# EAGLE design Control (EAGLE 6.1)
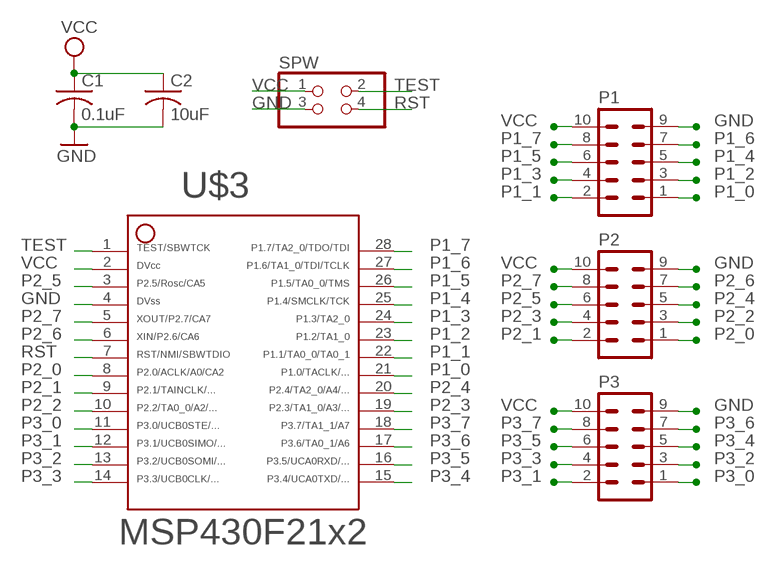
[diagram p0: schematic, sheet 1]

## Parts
C1  0.1uF  C-USC0603K  [C0603K]
C2  10uF  C-USC0603K  [C0603K]
P1  MA05-2  [MA05-2]
P2  MA05-2  [MA05-2]
P3  MA05-2  [MA05-2]
SPW  PINHD-2X2  [2X02]
U$3  F21X2---PW28  [PW28]

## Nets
GND: C1.2 C2.2 P1.9 P2.9 P3.9 SPW.3 U$3.4
P1_0: P1.1 U$3.21
P1_1: P1.2 U$3.22
P1_2: P1.3 U$3.23
P1_3: P1.4 U$3.24
P1_4: P1.5 U$3.25
P1_5: P1.6 U$3.26
P1_6: P1.7 U$3.27
P1_7: P1.8 U$3.28
P2_0: P2.1 U$3.8
P2_1: P2.2 U$3.9
P2_2: P2.3 U$3.10
P2_3: P2.4 U$3.19
P2_4: P2.5 U$3.20
P2_5: P2.6 U$3.3
P2_6: P2.7 U$3.6
P2_7: P2.8 U$3.5
P3_0: P3.1 U$3.11
P3_1: P3.2 U$3.12
P3_2: P3.3 U$3.13
P3_3: P3.4 U$3.14
P3_4: P3.5 U$3.15
P3_5: P3.6 U$3.16
P3_6: P3.7 U$3.17
P3_7: P3.8 U$3.18
RST: SPW.4 U$3.7
TEST: SPW.2 U$3.1
VCC: C1.1 C2.1 P1.10 P2.10 P3.10 SPW.1 U$3.2

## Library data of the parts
C1 C2 = rcl:C-US: CAPACITOR, American symbol
P1-P3 = con-lstb:MA05-2: PIN HEADER; OC_FARNELL: unknown; OC_NEWARK: unknown
SPW = pinhead:PINHD-2X2: PIN HEADER
U$3 = TI_MSP430_v16:F21X2---PW28: *** MSP430F21x2 *** PW28

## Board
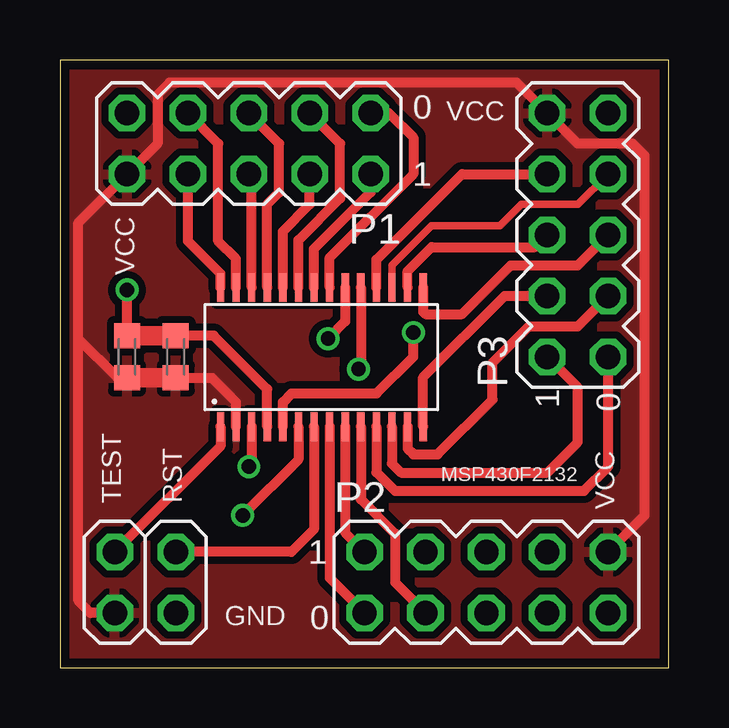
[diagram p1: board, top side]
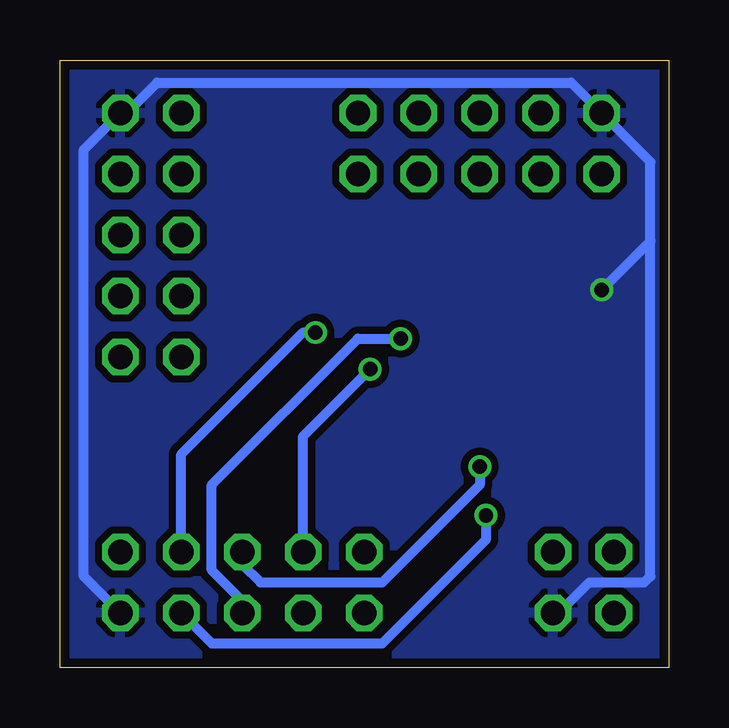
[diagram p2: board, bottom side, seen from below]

Size 25.38 x 25.32 mm. Coordinates in mm from the lower left corner, seen from the top.
Outline: 0,0 25.38,0 25.38,25.32 0,25.32 0,0
Copper layers (1*16): Top 0.0356mm / dielectric 1.5011mm / Bottom 0.0356mm
Design rules: minimum track width 6mil, minimum drill 13mil, track to track 6mil, track to pad 6mil, pad to pad 6mil, via to via 6mil, smd to smd 6mil, copper to edge 15mil, drill to drill 6mil, minimum pad ring 7mil, minimum via ring 7mil, stop-mask expansion 4mil, vias tented up to drill 0mil, thermal gap 10mil

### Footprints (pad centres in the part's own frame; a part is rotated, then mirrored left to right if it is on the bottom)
C0603K = smd 1.05 x 1.08: 1 -0.875,0; 2 0.875,0
MA05-2 = drill 1.016 octagon: 1 -5.08,-1.27; 2 -5.08,1.27; 3 -2.54,-1.27; 4 -2.54,1.27; 5 0,-1.27; 6 0,1.27; 7 2.54,-1.27; 8 2.54,1.27; 9 5.08,-1.27; 10 5.08,1.27
2X02 = drill 1.016 octagon: 1 -1.27,-1.27; 2 -1.27,1.27; 3 1.27,-1.27; 4 1.27,1.27
PW28 = smd 0.3 x 1.2: 1 -4.229,-2.908; 2 -3.579,-2.908; 3 -2.929,-2.908; 4 -2.279,-2.908; 5 -1.629,-2.908; 6 -0.979,-2.908; 7 -0.329,-2.908; 8 0.321,-2.908; 9 0.971,-2.908; 10 1.621,-2.908; 11 2.271,-2.908; 12 2.921,-2.908; 13 3.571,-2.908; 14 4.221,-2.908; 15 4.221,2.892; 16 3.571,2.892; 17 2.921,2.892; 18 2.271,2.892; 19 1.621,2.892; 20 0.971,2.892; 21 0.321,2.892; 22 -0.329,2.892; 23 -0.979,2.892; 24 -1.629,2.892; 25 -2.279,2.892; 26 -2.929,2.892; 27 -3.579,2.892; 28 -4.229,2.892

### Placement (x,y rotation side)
C1  4.83,12.95 90 top
C2  2.79,12.95 90 top
P1  7.87,21.84 180 top
P2  17.78,3.56 0 top
P3  21.59,18.03 90 top
SPW  3.56,3.56 0 top
U$3  10.92,12.95 0 top

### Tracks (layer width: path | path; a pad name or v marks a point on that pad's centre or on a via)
GND  (via drill 0.6)
  Top 0.406: U$3.4 8.64,11.61 6.41,13.84 4.84,13.84 C1.2 | C2.2 v2.79,15.75
  Top 0.813: C1.2 C2.2
  Bottom 0.406: P2.9 24.38,3.81 24.38,21.59 P3.9 22.61,23.11 21.34,24.38 4.06,24.38 P1.9 0.76,21.08 0.76,17.78 | SPW.3 4.57,2.29 3.3,3.56 1.02,3.56 0.76,3.81 0.76,17.78 | v2.79,15.75 0.76,17.78
  pour Bottom (isolate 0.305): 0,25.4 0,0 25.4,0 25.4,25.4
P1_0
  Top 0.406: U$3.21 11.24,17.09 14.73,20.57 14.73,22.1 13.72,23.11 P1.1
P1_1
  Top 0.406: U$3.22 10.59,17.45 12.95,19.81 P1.2
P1_2
  Top 0.406: P1.3 11.68,21.84 11.68,19.56 9.94,17.82 U$3.23
P1_3
  Top 0.406: U$3.24 9.29,18.18 10.41,19.3 P1.4
P1_4
  Top 0.406: U$3.25 8.64,19.31 9.14,19.81 9.14,21.84 P1.5
P1_5
  Top 0.406: U$3.26 7.99,20.45 P1.6
P1_6
  Top 0.406: U$3.27 7.34,17.04 6.6,17.78 6.6,21.84 P1.7
P1_7
  Top 0.406: U$3.28 6.69,16.42 5.33,17.78 P1.8
P2_0
  Top 0.406: U$3.8 11.24,3.74 P2.1
P2_1
  Top 0.406: U$3.9 11.89,5.63 P2.2
P2_2
  Top 0.406: U$3.10 12.54,7.01 13.97,5.59 13.97,3.56 P2.3
P2_3  (via drill 0.6)
  Top 0.406: U$3.19 12.54,12.54 v12.45,12.45
  Bottom 0.406: P2.4 15.24,9.65 v12.45,12.45
P2_4  (via drill 0.6)
  Top 0.406: U$3.20 11.89,14.43 v11.18,13.72
  Bottom 0.406: P2.5 17.78,2.79 19.05,4.06 19.05,7.62 12.95,13.72 v11.18,13.72
P2_5  (via drill 0.6)
  Top 0.406: U$3.3 7.99,8.5 v7.87,8.38
  Bottom 0.406: v7.87,8.38 7.87,7.62 11.94,3.56 17.02,3.56 17.78,4.32 P2.6
P2_6  (via drill 0.6)
  Top 0.406: U$3.6 9.94,8.67 v7.62,6.35
  Bottom 0.406: v7.62,6.35 7.62,5.33 11.94,1.02 19.05,1.02 P2.7
P2_7  (via drill 0.6)
  Top 0.406: U$3.5 9.29,11.07 9.65,11.43 13.21,11.43 14.73,12.95 v14.73,13.97
  Bottom 0.406: P2.8 20.32,8.89 15.24,13.97 v14.73,13.97
P3_0
  Top 0.406: U$3.11 13.19,8.14 13.97,7.37 21.84,7.37 22.86,8.38 P3.1
P3_1
  Top 0.406: U$3.12 13.84,8.51 14.22,8.13 20.32,8.13 21.59,9.4 21.59,11.68 P3.2
P3_2
  Top 0.406: U$3.13 14.49,9.13 14.73,8.89 15.75,8.89 18.03,11.18 18.03,12.7 19.56,14.22 21.59,14.22 P3.3
P3_3
  Top 0.406: U$3.14 15.14,12.1 18.54,15.49 P3.4
P3_4
  Top 0.406: U$3.15 15.14,14.83 15.24,14.73 16.76,14.73 18.8,16.76 21.59,16.76 P3.5
P3_5
  Top 0.406: U$3.16 14.49,16.52 15.49,17.53 19.81,17.53 P3.6
P3_6
  Top 0.305: U$3.17 13.84,16.76 15.49,18.41 18.35,18.41 19.24,19.3 21.59,19.3 P3.7
P3_7
  Top 0.406: U$3.18 13.19,17 16.76,20.57 P3.8
RST
  Top 0.406: U$3.7 10.59,5.77 9.65,4.83 SPW.4
TEST
  Top 0.406: U$3.1 6.69,9.23 SPW.2
VCC
  Top 0.406: SPW.1 1.27,2.29 0.76,2.79 0.76,13.72 | 0.76,13.72 0.76,18.54 P1.10 4.06,21.84 4.06,23.88 4.57,24.38 19.05,24.38 P3.10 21.59,21.84 23.88,21.84 24.38,21.34 24.38,6.35 P2.10 | U$3.2 7.34,11.07 6.35,12.06 4.84,12.06 C1.1 | C2.1 2.4,12.08 0.76,13.72
  Top 0.813: C1.1 C2.1
  pour Top (isolate 0.305): 0,0 0,25.4 25.4,25.4 25.4,0

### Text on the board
tPlace: VCC | VCC | MSP430F2132 | TEST | RST | VCC | GND
tNames: 0 | 1 | 1 | 0 | 1 | 0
